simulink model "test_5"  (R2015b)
settings: Solver=FixedStepDiscrete  StartTime=0.0  StopTime=10  RelTol=1e-3
undefined symbols (not defined in the file or in its folder): fir1

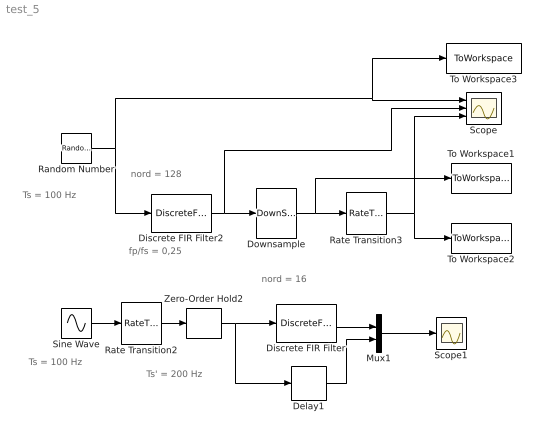
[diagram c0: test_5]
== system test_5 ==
  note: fp/fs = 0,25
  note: Ts = 100 Hz
  note: nord = 128
  note: nord = 16
  note: Ts' = 200 Hz
  note: Ts = 100 Hz
  Delay1 : Delay  DelayLength=8
  Discrete FIR Filter : DiscreteFir  Coefficients=fir1(16,0.01)
  Discrete FIR Filter2 : DiscreteFir  Coefficients=fir1(128,0.25)
  Downsample : DownSample  N=4  RateOptions=Allow multirate processing
  Mux1 : Mux  Inputs=2
  Random Number : RandomNumber  SampleTime=.01
  Rate Transition2 : RateTransition
  Rate Transition3 : RateTransition
  Scope : Scope  NumInputPorts=3
  Scope1 : Scope
  Sine Wave : Sin  Frequency=2*pi*0.5  SampleTime=0.01
  To Workspace1 : ToWorkspace  VariableName=y2  SaveFormat=Timeseries  SampleTime=-1
  To Workspace2 : ToWorkspace  VariableName=y3  SaveFormat=Timeseries  SampleTime=-1
  To Workspace3 : ToWorkspace  VariableName=y1  SaveFormat=Timeseries  SampleTime=-1
  Zero-Order Hold2 : ZeroOrderHold  SampleTime=0.005
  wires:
  Random Number/1 -> Scope/1, To Workspace3/1, Discrete FIR Filter2/1
  Discrete FIR Filter/1 -> Mux1/1
  Mux1/1 -> Scope1/1
  Delay1/1 -> Mux1/2
  Sine Wave/1 -> Rate Transition2/1
  Downsample/1 -> Rate Transition3/1, To Workspace1/1
  Discrete FIR Filter2/1 -> Scope/2, Downsample/1
  Zero-Order Hold2/1 -> Delay1/1, Discrete FIR Filter/1
  Rate Transition2/1 -> Zero-Order Hold2/1
  Rate Transition3/1 -> Scope/3, To Workspace2/1
